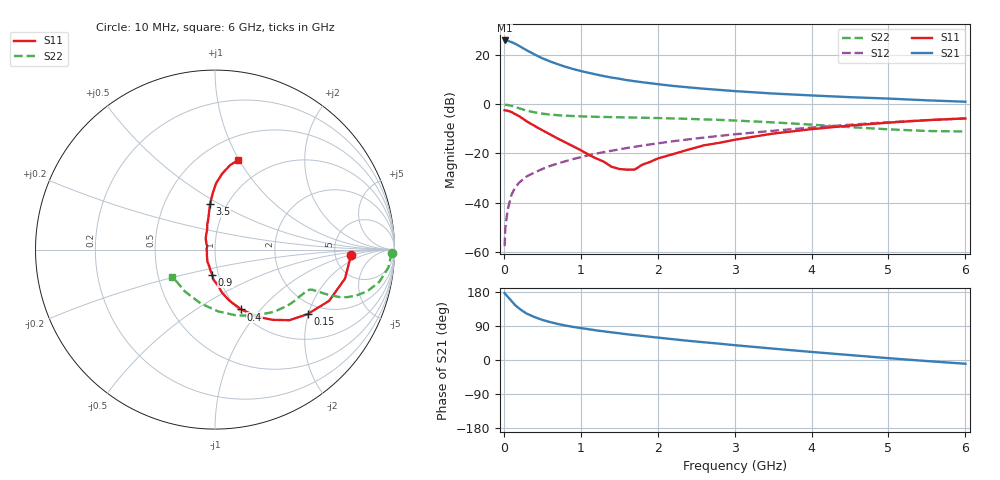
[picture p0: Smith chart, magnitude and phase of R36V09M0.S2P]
! SIEMENS Small Signal Semiconductors
! BFR181
! Si NPN RF Bipolar Junction Transistor in SOT23
! VCE = 6 V  IC = 9 mA
! Common Emitter S-Parameters:  May  1996
# GHz  S  MA  R  50
!  f  S11  S21  S12  S22
! GHz  MAG  ANG  MAG  ANG  MAG  ANG  MAG  ANG
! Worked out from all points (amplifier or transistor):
!   36 points, 10 MHz to 6 GHz, reference 50 ohm
!   highest |S21| = 26.0 dB at 10 MHz (marker M1)
!   |S21| within 3 dB of that: start of sweep to 241.8 MHz
!   unconditionally stable (mu >= 1): 886.1 MHz to 2.781 GHz
!   at 250 MHz: K = 0.57, MSG = 26.7 dB, |S12| = -30.5 dB
!   at 1.4 GHz: K = 1.05, MAG = 13.5 dB, |S12| = -18.9 dB
!   at 6 GHz: K = 0.86, MSG = 3.4 dB, |S12| = -5.7 dB
!   S11 on the Smith chart (normalised r, x): 10 MHz: 7.11, -1.06; 150 MHz: 1.67, -1.98; 400 MHz: 1.03, -0.79; 900 MHz: 0.93, -0.26; 3.5 GHz: 0.83, +0.45; 6 GHz: 0.73, +0.99
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0.01  0.7583 -2.4  19.97 176.7  0.0013 99.8  0.987 -1.1
0.02  0.752 -4.9  19.96 174.1  0.0031 89.5  0.9798 -2.4
0.05  0.7422 -12.6  19.67 167.0  0.0072 83.2  0.9713 -5.9
0.1  0.6969 -24.2  18.47 155.6  0.0145 80.0  0.9328 -11.1
0.15  0.6291 -34.8  17.06 144.1  0.0207 73.9  0.8813 -15.2
0.2  0.5722 -43.4  15.45 135.8  0.0256 71.8  0.8299 -17.9
0.25  0.5081 -50.4  13.89 128.4  0.0298 69.1  0.7854 -19.7
0.3  0.4487 -57.0  12.55 122.2  0.0343 69.0  0.7465 -20.8
0.4  0.3642 -66.3  10.36 113.2  0.0412 67.9  0.6862 -21.7
0.5  0.2972 -74.1  8.661 105.8  0.0483 68.2  0.6464 -22.0
0.6  0.2456 -80.4  7.486 100.2  0.0557 68.5  0.6208 -22.1
0.7  0.2016 -85.2  6.573 95.2  0.0626 69.0  0.6018 -22.3
0.9  0.1401 -96.6  5.236 87.3  0.077 68.9  0.5782 -22.7
1.1  0.095 -110.7  4.39 81.3  0.0918 69.0  0.5634 -24.0
1.3  0.0681 -129.7  3.756 75.6  0.1068 68.8  0.5535 -25.4
1.6  0.0468 174.7  3.113 67.9  0.1293 67.7  0.5418 -28.4
2.2  0.0972 120.3  2.371 54.8  0.1776 64.7  0.517 -35.8
3  0.1902 100.8  1.862 39.1  0.2455 58.8  0.469 -48.3
3.5  0.2543 96.3  1.661 30.0  0.2903 54.3  0.4296 -58.6
4.5  0.3704 89.0  1.4 13.0  0.3851 43.5  0.3442 -87.3
5.5  0.4765 80.0  1.207 -2.8  0.4773 31.1  0.2871 -125.9
6  0.5171 75.4  1.131 -9.9  0.5195 24.2  0.2806 -147.7
